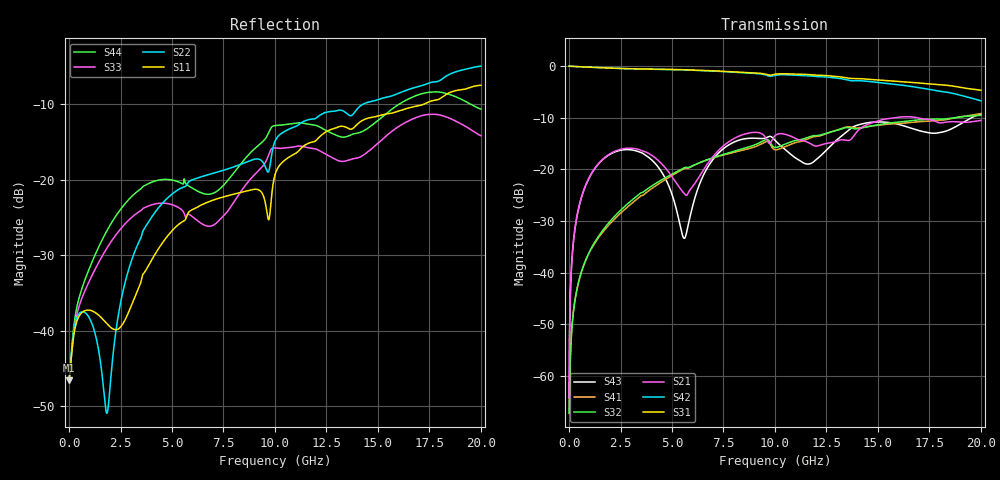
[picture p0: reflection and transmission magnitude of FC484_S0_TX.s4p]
! Touchstone generated by fitter/viewer
# HZ S  RI R 5.000000e+001
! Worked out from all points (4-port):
!   4999 points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, 4.001 MHz to 20 GHz, reference 50 ohm
!   strongest paths, dB at 4.001 MHz, 5.001 GHz, 10 GHz, 15 GHz, 20 GHz:
!     S31: 0.0, -0.7, -1.6, -2.7, -4.7
!     S42: 0.0, -0.7, -1.8, -3.2, -6.7
!     S21: -64.2, -21.4, -13.5, -10.6, -10.5
!     S32: -67.2, -20.9, -15.8, -11.4, -9.6
!     S41: -67.2, -21.2, -16.2, -11.5, -9.2
!     S43: -64.2, -24.8, -14.4, -10.8, -9.3
!   lowest |S11| = -46.6 dB at 4.001 MHz (marker M1), VSWR 1.01, Z = 50.5 + j0.0331 ohm
!   |S11| at or under -10 dB: start of sweep to 17.22 GHz
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4000800  0.00467 0.000327  0.00041 0.000465  0.9953 -0.00262  -0.000407 -0.000161
         0.00041 0.000465  0.00467 0.00035  -0.000407 -0.000161  0.9953 -0.00263
         0.9953 -0.00262  -0.000407 -0.000161  0.00467 0.00033  0.00041 0.000465
         -0.000407 -0.000161  0.9953 -0.00263  0.00041 0.000465  0.00467 0.000353
4.320864e8  0.0119 0.00181  0.0103 0.0382  0.9556 -0.2367  -0.00332 -0.00689
            0.0103 0.0382  0.0118 0.00443  -0.00314 -0.00697  0.9552 -0.2385
            0.9556 -0.2367  -0.00314 -0.00697  0.0135 0.00231  0.0118 0.0373
            -0.00332 -0.00689  0.9552 -0.2385  0.0118 0.0373  0.0147 0.00453
2.040408e9  -0.00249 -0.0102  0.1202 0.0786  0.4353 -0.8476  -0.0276 -0.0131
            0.1202 0.0786  -0.00109 0.00495  -0.0288 -0.0146  0.4272 -0.8516
            0.4353 -0.8476  -0.0288 -0.0146  0.0161 -0.0354  0.1329 0.0493
            -0.0276 -0.0131  0.4272 -0.8516  0.1329 0.0493  0.0277 -0.0431
5.477095e9  0.0285 0.0441  0.0622 -0.00317  -0.8915 -0.2305  -0.024 0.0962
            0.0622 -0.00317  0.0541 0.07  -0.0201 0.0989  -0.8943 -0.2061
            -0.8915 -0.2305  -0.0201 0.0989  -0.0617 0.0136  -0.0194 -0.0145
            -0.024 0.0962  -0.8943 -0.2061  -0.0194 -0.0145  -0.091 0.0253
8.469694e9  0.0829 0.00778  0.2099 0.0571  -0.2205 0.8387  0.1536 0.0115
            0.2099 0.0571  0.1218 0.0414  0.1589 0.0102  -0.178 0.8412
            -0.2205 0.8387  0.1589 0.0102  0.074 -0.0482  0.1966 -0.00537
            0.1536 0.0115  -0.178 0.8412  0.1966 -0.00537  0.1128 -0.0723
1.476295e10  0.1907 -0.1769  0.2515 -0.1318  0.1132 -0.7287  -0.2498 0.0832
             0.2515 -0.1318  0.2501 -0.2188  -0.2477 0.0926  0.0344 -0.701
             0.1132 -0.7287  -0.2477 0.0926  0.1623 -0.0197  0.2845 -0.0317
             -0.2498 0.0832  0.0344 -0.701  0.2845 -0.0317  0.2304 -0.0343
2e10  -0.0418 -0.4208  -0.1602 -0.2503  -0.3681 0.4521  0.3393 -0.0707
      -0.1602 -0.2503  -0.2335 -0.5156  0.3127 -0.1144  -0.2199 0.404
      -0.3681 0.4521  0.3127 -0.1144  -0.00565 0.1957  0.2099 0.2708
      0.3393 -0.0707  -0.2199 0.404  0.2099 0.2708  0.016 0.2936
